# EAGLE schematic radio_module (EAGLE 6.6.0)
AUTHOR: Joshua Adkins; REV: A; TITLE: Radio Module

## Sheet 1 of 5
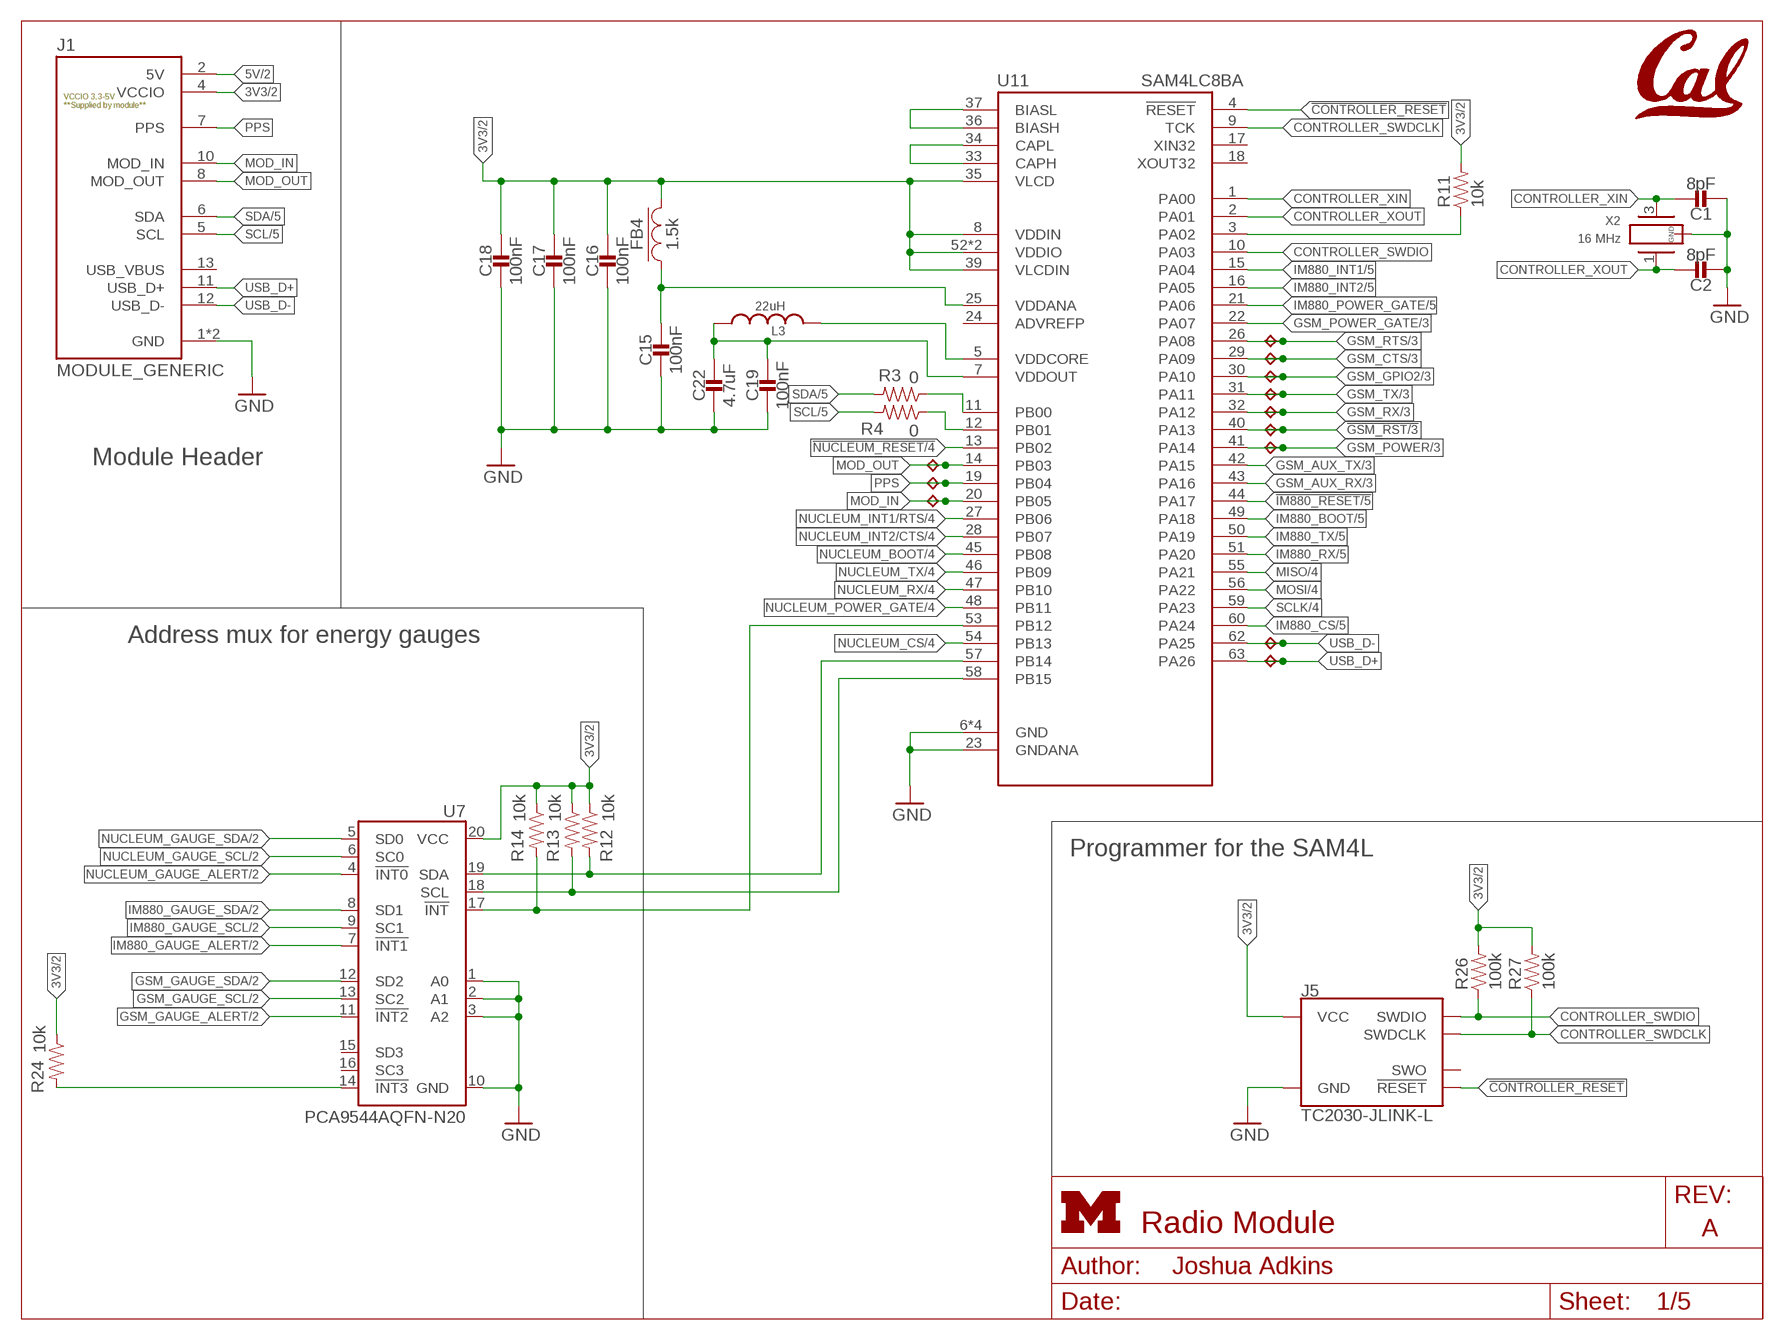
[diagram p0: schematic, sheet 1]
FRAME2 (LETTER_L_UMICH): HEIGHT: 8.5in; WIDTH: 11in

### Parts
C1  8pF  CAPACITOR0402_CAP  [0402_CAP]
C2  8pF  CAPACITOR0402_CAP  [0402_CAP]
C15  100nF  CAPACITOR0402_CAP  [0402_CAP]
C16  100nF  CAPACITOR0402_CAP  [0402_CAP]
C17  100nF  CAPACITOR0402_CAP  [0402_CAP]
C18  100nF  CAPACITOR0402_CAP  [0402_CAP]
C19  100nF  CAPACITOR0402_CAP  [0402_CAP]
C22  4.7uF  CAPACITOR0402_CAP  [0402_CAP]
FB4  1.5k  FERRITE_BEAD0402  [0402_CAP]
J1  MODULE_GENERIC  [MODULE_GENERIC]
J5  TC2030-JLINK-L  [TC2030-IDC]
L3  22uH  LHQ3NP  [1212]
R3  0  RESISTOR0402_RES  [0402_RES]
R4  0  RESISTOR0402_RES  [0402_RES]
R11  10k  RESISTOR0402_RES  [0402_RES]
R12  10k  RESISTOR0402_RES  [0402_RES]
R13  10k  RESISTOR0402_RES  [0402_RES]
R14  10k  RESISTOR0402_RES  [0402_RES]
R24  10k  RESISTOR0402_RES  [0402_RES]
R26  100k  RESISTOR0402_RES  [0402_RES]
R27  100k  RESISTOR0402_RES  [0402_RES]
TP1  TPB1,27  [B1,27]
TP2  TPB1,27  [B1,27]
TP3  TPB1,27  [B1,27]
TP4  TPB1,27  [B1,27]
TP5  TPB1,27  [B1,27]
TP6  TPB1,27  [B1,27]
TP7  TPB1,27  [B1,27]
TP8  TPB1,27  [B1,27]
TP9  TPB1,27  [B1,27]
TP10  TPB1,27  [B1,27]
TP11  TPB1,27  [B1,27]
TP12  TPB1,27  [B1,27]
U7  PCA9544AQFN-N20  [QFN-N20]
U11  SAM4LC8BA  [QFN-64-9MM]
U$1  UCB_CAL100MIL  [UCB_CAL_100MIL]
X2  16 MHz  FH1600015  [FHXXX]

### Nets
3V3: C16.1 C17.1 C18.1 FB4.2 J1.4(VCCIO) J5.1(VCC) R11.2 R12.1 R13.1 R14.1 R24.1 R26.2 R27.2 U7.20(VCC) U11.8(VDDIN) U11.35(VLCD) U11.39(VLCDIN) U11.52(VDDIO) U11.61(VDDIO) ; also sheet 2,3
5V: J1.2(5V) ; also sheet 2
!CONTROLLER_RESET: J5.3(!RESET) U11.4(!RESET)
!GSM_RST: TP7.TP U11.40(PA13) ; also sheet 3
!IM880_RESET: U11.44(PA17) ; also sheet 5
!NUCLEUM_RESET: U11.13(PB02) ; also sheet 4
CONTROLLER_BUCK/LDO_N: R11.1 U11.3(PA02)
CONTROLLER_SWDCLK: J5.4(SWDCLK) R27.1 U11.9(TCK)
CONTROLLER_SWDIO: J5.2(SWDIO) R26.1 U11.10(PA03)
CONTROLLER_XIN: C1.1 U11.1(PA00) X2.3
CONTROLLER_XOUT: C2.1 U11.2(PA01) X2.1
GND: C1.2 C2.2 C15.2 C16.2 C17.2 C18.2 C19.2 C22.2 J1.1(GND) J1.14(GND) J5.5(GND) U7.1(A0) U7.2(A1) U7.3(A2) U7.10(GND) U11.6(GND) U11.23(GNDANA) U11.38(GND) U11.64(GND) U11.GND X2.2(GND) X2.4(GND) ; also sheet 2,3,4,5
GSM_AUX_RX: U11.43(PA16) ; also sheet 3
GSM_AUX_TX: U11.42(PA15) ; also sheet 3
GSM_CTS: TP11.TP U11.29(PA09) ; also sheet 3
GSM_GAUGE_ALERT: U7.11(!INT2) ; also sheet 2
GSM_GAUGE_SCL: U7.13(SC2) ; also sheet 2
GSM_GAUGE_SDA: U7.12(SD2) ; also sheet 2
GSM_GPIO2: TP10.TP U11.30(PA10) ; also sheet 3
GSM_POWER: TP6.TP U11.41(PA14) ; also sheet 3
GSM_POWER_GATE: U11.22(PA07) ; also sheet 3
GSM_RTS: TP12.TP U11.26(PA08) ; also sheet 3
GSM_RX: TP8.TP U11.32(PA12) ; also sheet 3
GSM_TX: TP9.TP U11.31(PA11) ; also sheet 3
IM880_BOOT: U11.49(PA18) ; also sheet 5
IM880_CS: U11.60(PA24) ; also sheet 5
IM880_GAUGE_ALERT: U7.7(!INT1) ; also sheet 2
IM880_GAUGE_SCL: U7.9(SC1) ; also sheet 2
IM880_GAUGE_SDA: U7.8(SD1) ; also sheet 2
IM880_INT1: U11.15(PA04) ; also sheet 5
IM880_INT2: U11.16(PA05) ; also sheet 5
IM880_POWER_GATE: U11.21(PA06) ; also sheet 5
IM880_RX: U11.51(PA20) ; also sheet 5
IM880_TX: U11.50(PA19) ; also sheet 5
MISO: U11.55(PA21) ; also sheet 4,5
MOD_IN: J1.10(MOD_IN) TP3.TP U11.20(PB05)
MOD_OUT: J1.8(MOD_OUT) TP1.TP U11.14(PB03)
MOSI: U11.56(PA22) ; also sheet 4,5
N$9: R14.2 U7.17(!INT) U11.53(PB12)
N$12: R24.2 U7.14(!INT3)
N$17: R3.1 U11.11(PB00)
N$18: R4.1 U11.12(PB01)
N$33: C15.1 FB4.1 U11.25(VDDANA)
N$44: C19.1 C22.1 L3.P$1 U11.7(VDDOUT)
N$52: L3.P$2 U11.5(VDDCORE)
N$53: U11.36(BIASH) U11.37(BIASL)
N$54: U11.33(CAPH) U11.34(CAPL)
NUCLEUM_BOOT: U11.45(PB08) ; also sheet 4
NUCLEUM_CS: U11.54(PB13) ; also sheet 4
NUCLEUM_GAUGE_ALERT: U7.4(!INT0) ; also sheet 2
NUCLEUM_GAUGE_SCL: U7.6(SC0) ; also sheet 2
NUCLEUM_GAUGE_SDA: U7.5(SD0) ; also sheet 2
NUCLEUM_INT1/RTS: U11.27(PB06) ; also sheet 4
NUCLEUM_INT2/CTS: U11.28(PB07) ; also sheet 4
NUCLEUM_POWER_GATE: U11.48(PB11) ; also sheet 4
NUCLEUM_RX: U11.47(PB10) ; also sheet 4
NUCLEUM_TX: U11.46(PB09) ; also sheet 4
PPS: J1.7(PPS) TP2.TP U11.19(PB04)
SCL: J1.5(SCL) R4.2 ; also sheet 5
SCL_INTERNAL: R13.2 U7.18(SCL) U11.58(PB15)
SCLK: U11.59(PA23) ; also sheet 4,5
SDA: J1.6(SDA) R3.2 ; also sheet 5
SDA_INTERNAL: R12.2 U7.19(SDA) U11.57(PB14)
USB_D+: J1.11(USB_D+) TP4.TP U11.63(PA26)
USB_D-: J1.12(USB_D-) TP5.TP U11.62(PA25)
Unconnected: J1.13(USB_VBUS) J5.6(SWO) U7.15(SD3) U7.16(SC3) U11.17(XIN32) U11.18(XOUT32)

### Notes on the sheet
- Module Header
- Address mux for energy gauges
- Programmer for the SAM4L

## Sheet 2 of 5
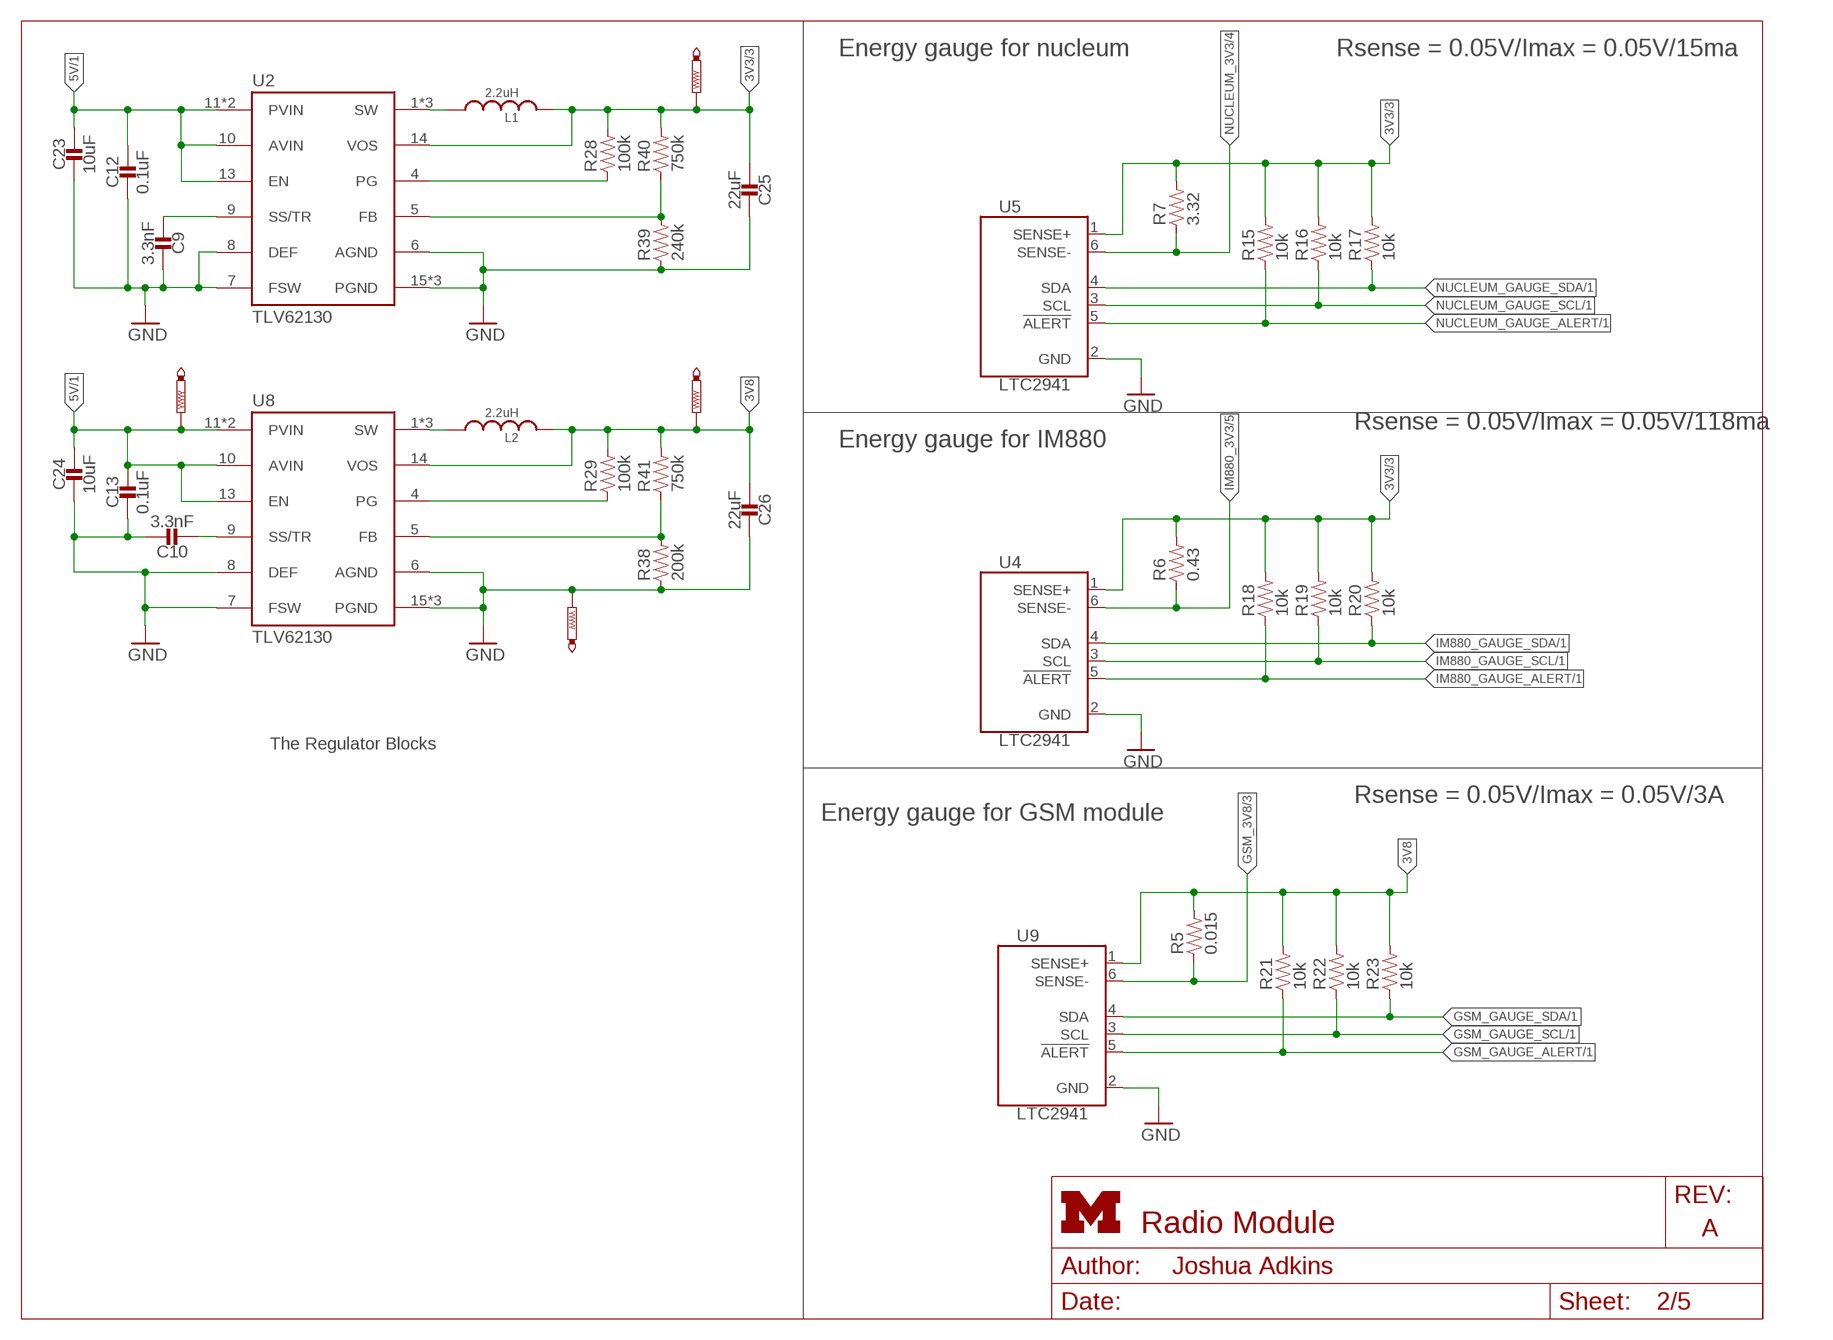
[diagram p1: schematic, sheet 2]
FRAME5 (LETTER_L_UMICH): HEIGHT: 8.5in; WIDTH: 11in

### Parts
C9  3.3nF  CAPACITOR0402_CAP  [0402_CAP]
C10  3.3nF  CAPACITOR0402_CAP  [0402_CAP]
C12  0.1uF  CAPACITOR0402_CAP  [0402_CAP]
C13  0.1uF  CAPACITOR0402_CAP  [0402_CAP]
C23  10uF  CAPACITOR0402_CAP  [0402_CAP]
C24  10uF  CAPACITOR0402_CAP  [0402_CAP]
C25  22uF  CAPACITOR0402_CAP  [0402_CAP]
C26  22uF  CAPACITOR0402_CAP  [0402_CAP]
L1  2.2uH  INDUCTORIHL  [IHL-1212BZ-11]
L2  2.2uH  INDUCTORIHL  [IHL-1212BZ-11]
R5  0.015  RESISTOR0603_RES  [0603-RES]
R6  0.43  RESISTOR0402_RES  [0402_RES]
R7  3.32  RESISTOR0402_RES  [0402_RES]
R15  10k  RESISTOR0402_RES  [0402_RES]
R16  10k  RESISTOR0402_RES  [0402_RES]
R17  10k  RESISTOR0402_RES  [0402_RES]
R18  10k  RESISTOR0402_RES  [0402_RES]
R19  10k  RESISTOR0402_RES  [0402_RES]
R20  10k  RESISTOR0402_RES  [0402_RES]
R21  10k  RESISTOR0402_RES  [0402_RES]
R22  10k  RESISTOR0402_RES  [0402_RES]
R23  10k  RESISTOR0402_RES  [0402_RES]
R28  100k  RESISTOR0402_RES  [0402_RES]
R29  100k  RESISTOR0402_RES  [0402_RES]
R38  200k  RESISTOR0402_RES  [0402_RES]
R39  240k  RESISTOR0402_RES  [0402_RES]
R40  750k  RESISTOR0402_RES  [0402_RES]
R41  750k  RESISTOR0402_RES  [0402_RES]
TP14  PTR1PAD1-13  [P1-13]
TP15  PTR1PAD1-13  [P1-13]
TP16  PTR1PAD1-13  [P1-13]
TP17  PTR1PAD1-13  [P1-13]
U2  TLV62130  [TQFN-16/3MM]
U4  LTC2941  [DFN-6-2MMX3MM]
U5  LTC2941  [DFN-6-2MMX3MM]
U8  TLV62130  [TQFN-16/3MM]
U9  LTC2941  [DFN-6-2MMX3MM]

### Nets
3V3: C25.2 L1.P$2 R6.2 R7.2 R15.2 R16.2 R17.2 R18.2 R19.2 R20.2 R28.2 R40.2 TP17.TP U2.14(VOS) U4.1(SENSE+) U5.1(SENSE+) ; also sheet 1,3
3V8: C26.2 L2.P$2 R5.2 R21.2 R22.2 R23.2 R29.2 R41.2 TP14.TP U8.14(VOS) U9.1(SENSE+)
3V8SWOUT: L2.P$1 U8.1(SW) U8.2(SW) U8.3(SW)
3VSWOUT: L1.P$1 U2.1(SW) U2.2(SW) U2.3(SW)
5V: C12.1 C13.1 C23.1 C24.1 TP16.TP U2.10(AVIN) U2.11(PVIN) U2.12(PVIN) U2.13(EN) U8.10(AVIN) U8.11(PVIN) U8.12(PVIN) U8.13(EN) ; also sheet 1
GND: C9.1 C10.1 C12.2 C13.2 C23.2 C24.2 C25.1 C26.1 R38.1 R39.1 TP15.TP U2.6(AGND) U2.7(FSW) U2.8(DEF) U2.15(PGND) U2.16(PGND) U2.GND U4.2(GND) U5.2(GND) U8.6(AGND) U8.7(FSW) U8.8(DEF) U8.15(PGND) U8.16(PGND) U8.GND U9.2(GND) ; also sheet 1,3,4,5
GSM_3V8: R5.1 U9.6(SENSE-) ; also sheet 3
GSM_GAUGE_ALERT: R21.1 U9.5(!ALERT) ; also sheet 1
GSM_GAUGE_SCL: R22.1 U9.3(SCL) ; also sheet 1
GSM_GAUGE_SDA: R23.1 U9.4(SDA) ; also sheet 1
IM880_3V3: R6.1 U4.6(SENSE-) ; also sheet 5
IM880_GAUGE_ALERT: R18.1 U4.5(!ALERT) ; also sheet 1
IM880_GAUGE_SCL: R19.1 U4.3(SCL) ; also sheet 1
IM880_GAUGE_SDA: R20.1 U4.4(SDA) ; also sheet 1
N$34: C9.2 U2.9(SS/TR)
N$36: R28.1 U2.4(PG)
N$37: R39.2 R40.1 U2.5(FB)
N$38: C10.2 U8.9(SS/TR)
N$40: R29.1 U8.4(PG)
N$41: R38.2 R41.1 U8.5(FB)
NUCLEUM_3V3: R7.1 U5.6(SENSE-) ; also sheet 4
NUCLEUM_GAUGE_ALERT: R15.1 U5.5(!ALERT) ; also sheet 1
NUCLEUM_GAUGE_SCL: R16.1 U5.3(SCL) ; also sheet 1
NUCLEUM_GAUGE_SDA: R17.1 U5.4(SDA) ; also sheet 1

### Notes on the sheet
- Energy gauge for nucleum | Rsense = 0.05V/Imax = 0.05V/15ma
- Rsense = 0.05V/Imax = 0.05V/118ma
- Energy gauge for IM880
- The Regulator Blocks
- Rsense = 0.05V/Imax = 0.05V/3A
- Energy gauge for GSM module

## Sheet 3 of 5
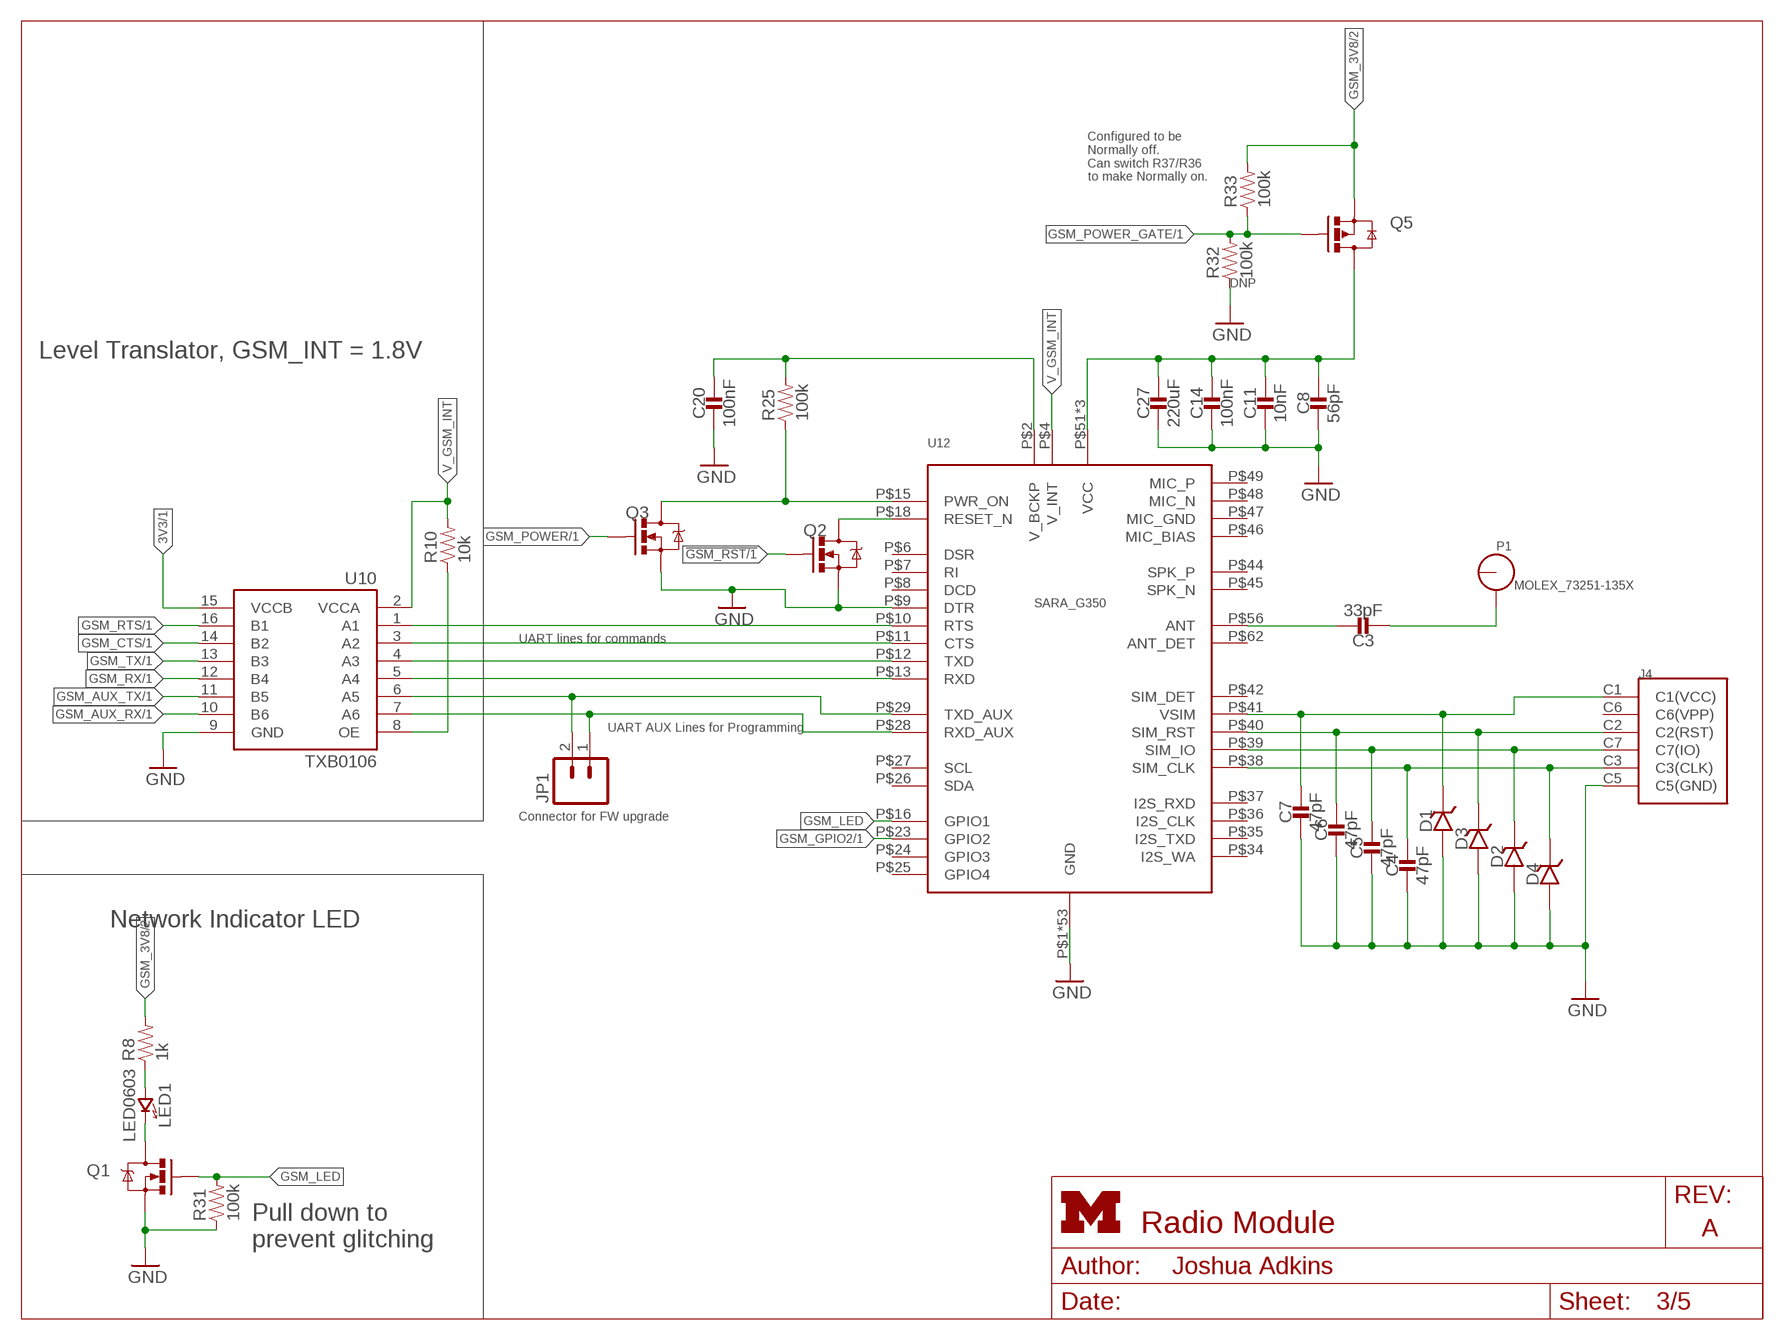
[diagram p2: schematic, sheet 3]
FRAME1 (LETTER_L_UMICH): HEIGHT: 8.5in; WIDTH: 11in

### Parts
C3  33pF  CAPACITOR0603_CAP  [0603_CAP]
C4  47pF  CAPACITOR0402_CAP  [0402_CAP]
C5  47pF  CAPACITOR0402_CAP  [0402_CAP]
C6  47pF  CAPACITOR0402_CAP  [0402_CAP]
C7  47pF  CAPACITOR0402_CAP  [0402_CAP]
C8  56pF  CAPACITOR0402_CAP  [0402_CAP]
C11  10nF  CAPACITOR0402_CAP  [0402_CAP]
C14  100nF  CAPACITOR0402_CAP  [0402_CAP]
C20  100nF  CAPACITOR0402_CAP  [0402_CAP]
C27  220uF  CAPACITOR1210_CAP  [1210_CAP]
D1  14V  DIODE_ZENER  [0402_DIODE]
D2  DIODE_ZENER  [0402_DIODE]
D3  DIODE_ZENER  [0402_DIODE]
D4  DIODE_ZENER  [0402_DIODE]
J4  NANO_SIM  [WURTH_NANO_SIM]
JP1  M02PTH  [1X02]
LED1  LED0603  [LED-0603]
P1  MOLEX_73251-135X  [SMA-J/PCB]
Q1  MOSFET-NCHANNELXFDN-3  [XFDFN-3]
Q2  MOSFET-NCHANNELXFDN-3  [XFDFN-3]
Q3  MOSFET-NCHANNELXFDN-3  [XFDFN-3]
Q5  SI223DDS  [SOT23-3]
R8  1k  RESISTOR0402_RES  [0402_RES]
R10  10k  RESISTOR0402_RES  [0402_RES]
R25  100k  RESISTOR0402_RES  [0402_RES]
R31  100k  RESISTOR0402_RES  [0402_RES]
R32  100k  RESISTOR0402_RES  [0402_RES]
R33  100k  RESISTOR0402_RES  [0402_RES]
U10  TXB0106  [R-PVQFN-N16]
U12  UBLOX_SARA_G350  [UBLOX_SARA_G3]

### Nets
3V3: U10.15(VCCB) ; also sheet 1,2
!GSM_RST: Q2.G ; also sheet 1
GND: C4.2 C5.2 C6.2 C7.2 C8.2 C11.2 C14.2 C20.2 C27.2 D1.ANODE D2.ANODE D3.ANODE D4.ANODE J4.C5(C5(GND)) Q1.S Q2.S Q3.S R31.1 R32.1 U10.9(GND) U12.P65(GND) U12.P66(GND) U12.P67(GND) U12.P68(GND) U12.P69(GND) U12.P70(GND) U12.P71(GND) U12.P72(GND) U12.P73(GND) U12.P74(GND) U12.P75(GND) U12.P76(GND) U12.P77(GND) U12.P78(GND) U12.P79(GND) U12.P80(GND) U12.P81(GND) U12.P82(GND) U12.P83(GND) U12.P84(GND) U12.P85(GND) U12.P86(GND) U12.P87(GND) U12.P88(GND) U12.P89(GND) U12.P90(GND) U12.P91(GND) U12.P92(GND) U12.P93(GND) U12.P94(GND) U12.P95(GND) U12.P96(GND) U12.P$1(GND) U12.P$3(GND) U12.P$5(GND) U12.P$9(DTR) U12.P$14(GND) U12.P$20(GND) U12.P$21(GND) U12.P$22(GND) U12.P$30(GND) U12.P$32(GND) U12.P$33(GND) U12.P$43(GND) U12.P$50(GND) U12.P$54(GND) U12.P$55(GND) U12.P$57(GND) U12.P$58(GND) U12.P$59(GND) U12.P$60(GND) U12.P$61(GND) U12.P$63(GND) U12.P$64(GND) ; also sheet 1,2,4,5
GSM_3V8: Q5.2(S) R8.2 R33.2 ; also sheet 2
GSM_AUX_RX: U10.10(B6) ; also sheet 1
GSM_AUX_TX: U10.11(B5) ; also sheet 1
GSM_CTS: U10.14(B2) ; also sheet 1
GSM_GATED: C8.1 C11.1 C14.1 C27.1 Q5.3(D) U12.P$51(VCC) U12.P$52(VCC) U12.P$53(VCC)
GSM_GPIO2: U12.P$23(GPIO2) ; also sheet 1
GSM_LED: Q1.G R31.2 U12.P$16(GPIO1)
GSM_POWER: Q3.G ; also sheet 1
GSM_POWER_GATE: Q5.1(G) R32.2 R33.1 ; also sheet 1
GSM_RTS: U10.16(B1) ; also sheet 1
GSM_RX: U10.12(B4) ; also sheet 1
GSM_TX: U10.13(B3) ; also sheet 1
N$1: C7.1 D1.CATHODE J4.C1(C1(VCC)) U12.P$41(VSIM)
N$2: C6.1 D3.CATHODE J4.C2(C2(RST)) U12.P$40(SIM_RST)
N$3: C5.1 D2.CATHODE J4.C7(C7(IO)) U12.P$39(SIM_IO)
N$4: C4.1 D4.CATHODE J4.C3(C3(CLK)) U12.P$38(SIM_CLK)
N$5: R10.1 U10.8(OE)
N$6: C3.1 U12.P$56(ANT)
N$7: C3.2 P1.2 P1.3 P1.4 P1.5
N$8: LED1.A(ANODE) R8.1
N$10: U10.4(A3) U12.P$12(TXD)
N$11: U10.5(A4) U12.P$13(RXD)
N$13: LED1.C(CATHODE) Q1.D
N$14: Q2.D U12.P$18(RESET_N)
N$15: C20.1 R25.2 U12.P$2(V_BCKP)
N$16: Q3.D R25.1 U12.P$15(PWR_ON)
N$20: JP1.2 U10.6(A5) U12.P$29(TXD_AUX)
N$21: JP1.1 U10.7(A6) U12.P$28(RXD_AUX)
N$22: U10.3(A2) U12.P$11(CTS)
N$23: U10.1(A1) U12.P$10(RTS)
V_GSM_INT: R10.2 U10.2(VCCA) U12.P$4(V_INT)
Unconnected: J4.C6(C6(VPP)) P1.1(ANT) U12.P$6(DSR) U12.P$7(RI) U12.P$8(DCD) U12.P$24(GPIO3) U12.P$25(GPIO4) U12.P$26(SDA) U12.P$27(SCL) U12.P$34(I2S_WA) U12.P$35(I2S_TXD) U12.P$36(I2S_CLK) U12.P$37(I2S_RXD) U12.P$42(SIM_DET) U12.P$44(SPK_P) U12.P$45(SPK_N) U12.P$46(MIC_BIAS) U12.P$47(MIC_GND) U12.P$48(MIC_N) U12.P$49(MIC_P) U12.P$62(ANT_DET)

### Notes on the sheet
- Configured to be
  Normally off.
  Can switch R37/R36 
  to make Normally on.
- DNP
- Level Translator, GSM_INT = 1.8V
- UART lines for commands
- UART AUX Lines for Programming
- Connector for FW upgrade
- Network Indicator LED
- Pull down to 
  prevent glitching

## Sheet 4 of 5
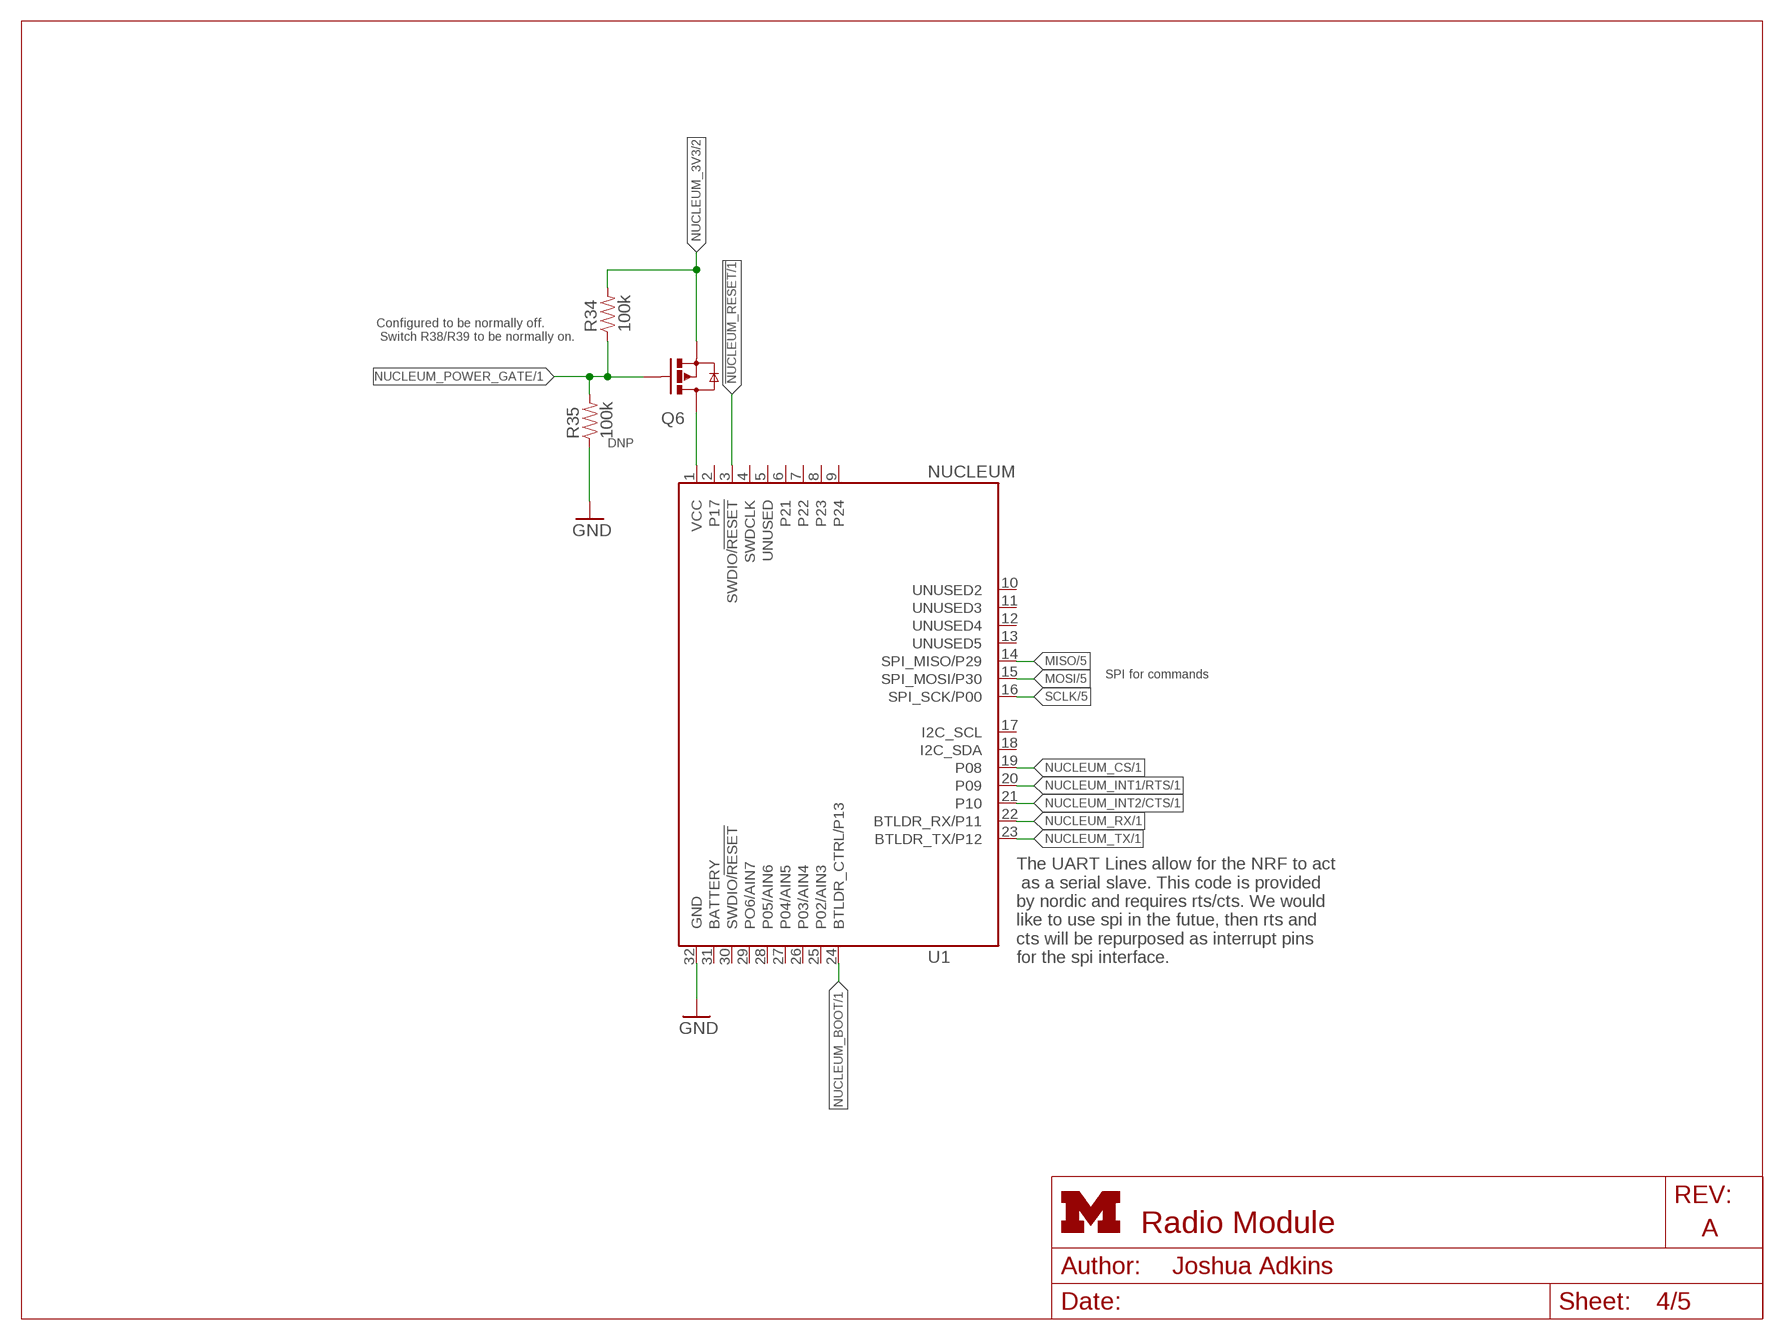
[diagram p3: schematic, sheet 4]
FRAME3 (LETTER_L_UMICH): HEIGHT: 8.5in; WIDTH: 11in

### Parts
Q6  SI223DDS  [SOT23-3]
R34  100k  RESISTOR0402_RES  [0402_RES]
R35  100k  RESISTOR0402_RES  [0402_RES]
U1  NUCLEUM  [NUCLEUM]

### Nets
!NUCLEUM_RESET: U1.3(SWDIO/!RESET) ; also sheet 1
GND: R35.1 U1.32(GND) ; also sheet 1,2,3,5
MISO: U1.14(SPI_MISO/P29) ; also sheet 1,5
MOSI: U1.15(SPI_MOSI/P30) ; also sheet 1,5
N$19: Q6.3(D) U1.1(VCC)
NUCLEUM_3V3: Q6.2(S) R34.2 ; also sheet 2
NUCLEUM_BOOT: U1.24(BTLDR_CTRL/P13) ; also sheet 1
NUCLEUM_CS: U1.19(P08) ; also sheet 1
NUCLEUM_INT1/RTS: U1.20(P09) ; also sheet 1
NUCLEUM_INT2/CTS: U1.21(P10) ; also sheet 1
NUCLEUM_POWER_GATE: Q6.1(G) R34.1 R35.2 ; also sheet 1
NUCLEUM_RX: U1.22(BTLDR_RX/P11) ; also sheet 1
NUCLEUM_TX: U1.23(BTLDR_TX/P12) ; also sheet 1
SCLK: U1.16(SPI_SCK/P00) ; also sheet 1,5
Unconnected: U1.2(P17) U1.4(SWDCLK) U1.5(UNUSED) U1.6(P21) U1.7(P22) U1.8(P23) U1.9(P24) U1.10(UNUSED2) U1.11(UNUSED3) U1.12(UNUSED4) U1.13(UNUSED5) U1.17(I2C_SCL) U1.18(I2C_SDA) U1.25(P02/AIN3) U1.26(P03/AIN4) U1.27(P04/AIN5) U1.28(P05/AIN6) U1.29(PO6/AIN7) U1.30(SWDIO/!RESET) U1.31(BATTERY)

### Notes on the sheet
- Configured to be normally off.
   Switch R38/R39 to be normally on.
- DNP
- SPI for commands
- The UART Lines allow for the NRF to act
   as a serial slave. This code is provided 
  by nordic and requires rts/cts. We would 
  like to use spi in the futue, then rts and 
  cts will be repurposed as interrupt pins 
  for the spi interface.

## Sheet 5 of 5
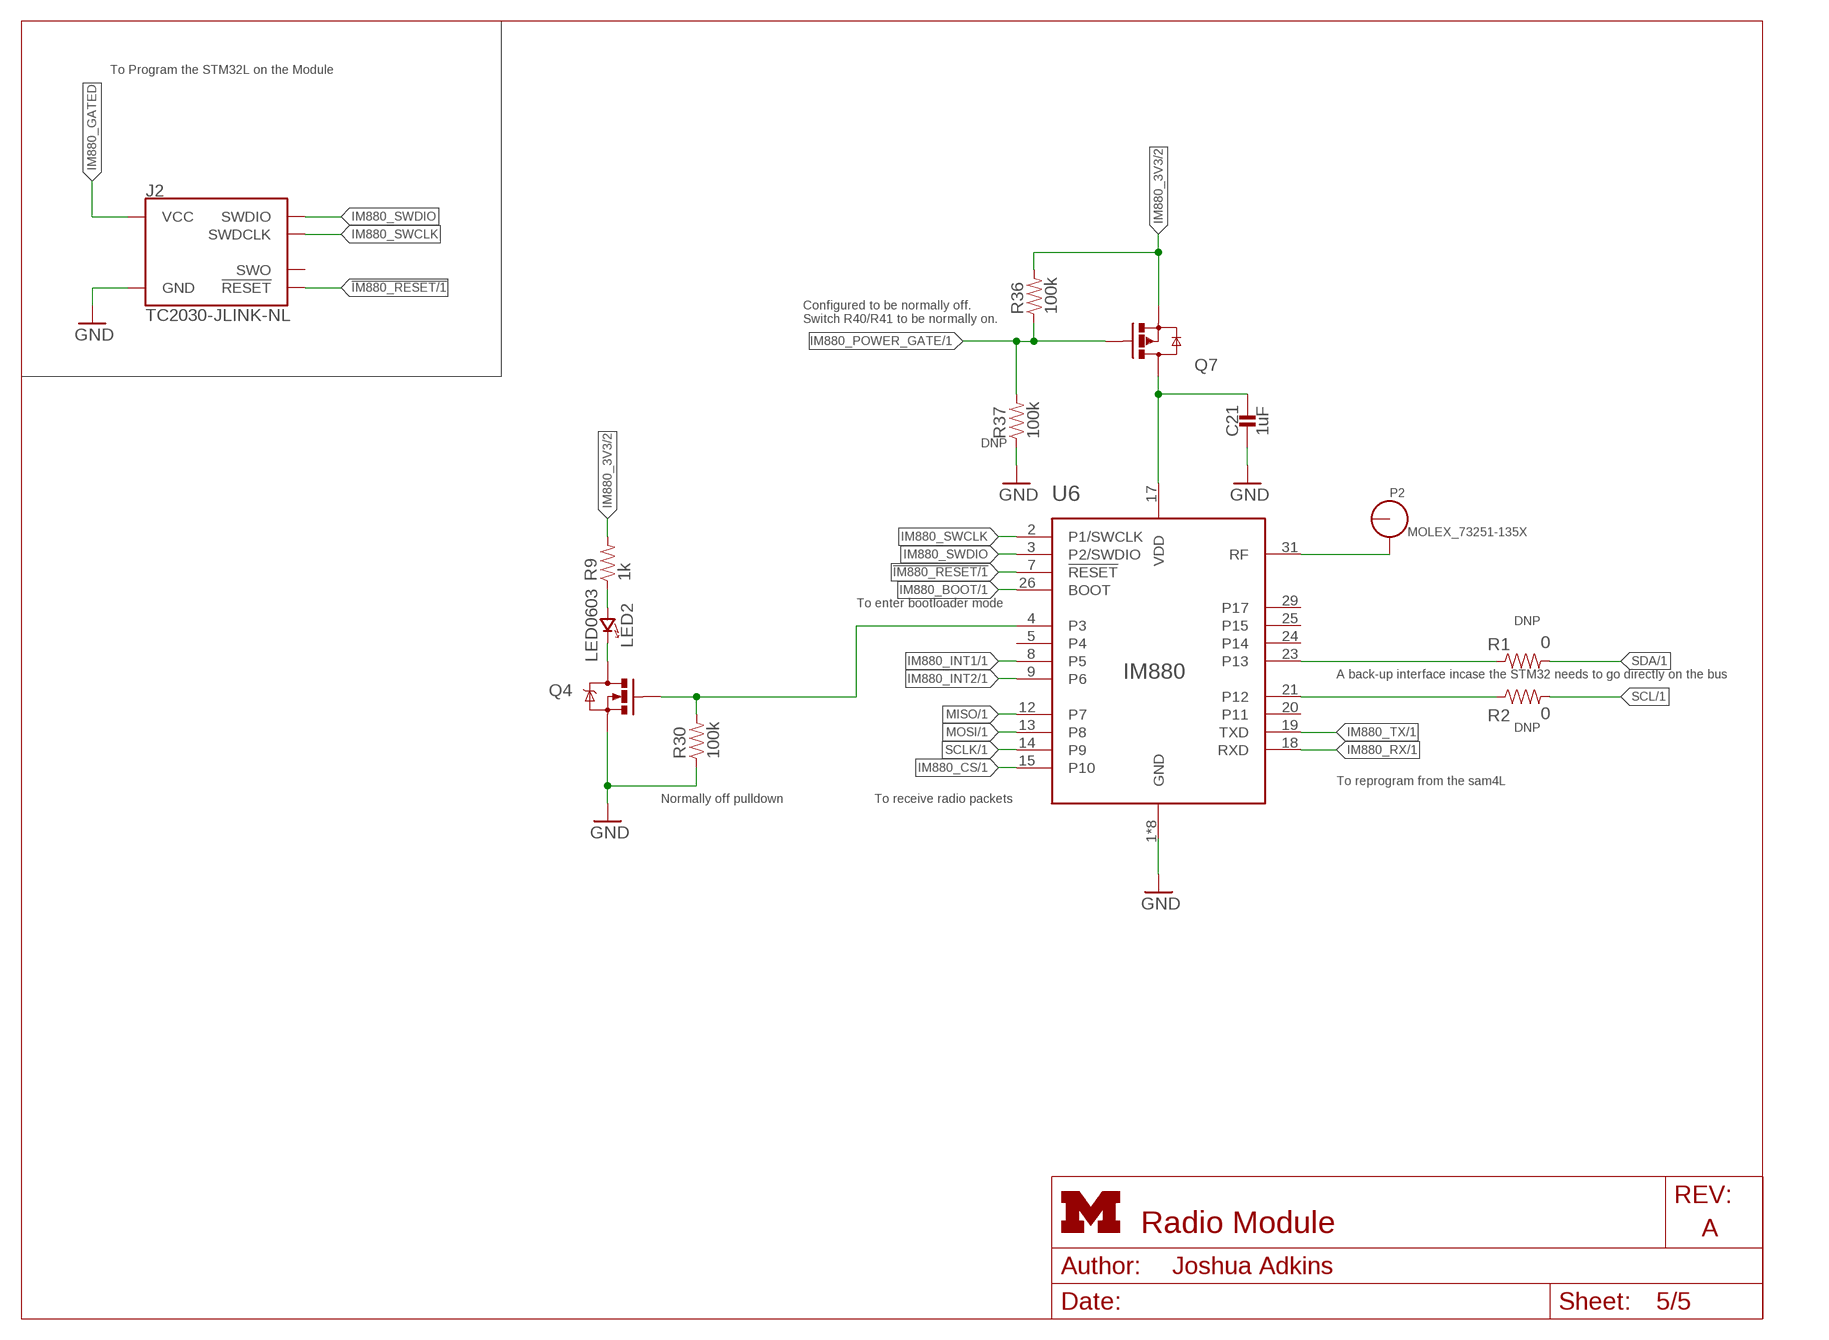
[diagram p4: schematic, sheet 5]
FRAME4 (LETTER_L_UMICH): HEIGHT: 8.5in; WIDTH: 11in

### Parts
C21  1uF  CAPACITOR0402_CAP  [0402_CAP]
J2  TC2030-JLINK-NL  [TC2030-IDC-NL]
LED2  LED0603  [LED-0603]
P2  MOLEX_73251-135X  [SMA-J/PCB]
Q4  MOSFET-NCHANNELXFDN-3  [XFDFN-3]
Q7  SI223DDS  [SOT23-3]
R1  0  RESISTOR0402_RES  [0402_RES]
R2  0  RESISTOR0402_RES  [0402_RES]
R9  1k  RESISTOR0402_RES  [0402_RES]
R30  100k  RESISTOR0402_RES  [0402_RES]
R36  100k  RESISTOR0402_RES  [0402_RES]
R37  100k  RESISTOR0402_RES  [0402_RES]
U6  IM880_MODULE  [IM880_MODULE]

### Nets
!IM880_RESET: J2.3(!RESET) U6.7(!RESET) ; also sheet 1
GND: C21.2 J2.5(GND) Q4.S R30.1 R37.1 U6.1(GND) U6.6(GND) U6.11(GND) U6.16(GND) U6.22(GND) U6.27(GND) U6.30(GND) U6.32(GND) ; also sheet 1,2,3,4
IM880_3V3: Q7.2(S) R9.2 R36.2 ; also sheet 2
IM880_BOOT: U6.26(BOOT) ; also sheet 1
IM880_CS: U6.15(P10) ; also sheet 1
IM880_GATED: C21.1 J2.1(VCC) Q7.3(D) U6.17(VDD)
IM880_INT1: U6.8(P5) ; also sheet 1
IM880_INT2: U6.9(P6) ; also sheet 1
IM880_NETWORK: Q4.G R30.2 U6.4(P3)
IM880_POWER_GATE: Q7.1(G) R36.1 R37.2 ; also sheet 1
IM880_RX: U6.18(RXD) ; also sheet 1
IM880_SWCLK: J2.4(SWDCLK) U6.2(P1/SWCLK)
IM880_SWDIO: J2.2(SWDIO) U6.3(P2/SWDIO)
IM880_TX: U6.19(TXD) ; also sheet 1
MISO: U6.12(P7) ; also sheet 1,4
MOSI: U6.13(P8) ; also sheet 1,4
N$25: R1.1 U6.23(P13)
N$26: R2.1 U6.21(P12)
N$27: LED2.A(ANODE) R9.1
N$28: LED2.C(CATHODE) Q4.D
N$29: P2.2 P2.3 P2.4 P2.5 U6.31(RF)
SCL: R2.2 ; also sheet 1
SCLK: U6.14(P9) ; also sheet 1,4
SDA: R1.2 ; also sheet 1
Unconnected: J2.6(SWO) P2.1(ANT) U6.5(P4) U6.20(P11) U6.24(P14) U6.25(P15) U6.29(P17)

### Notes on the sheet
- To Program the STM32L on the Module
- Configured to be normally off.
  Switch R40/R41 to be normally on.
- DNP
- To enter bootloader mode
- DNP
- A back-up interface incase the STM32 needs to go directly on the bus
- DNP
- To reprogram from the sam4L
- Normally off pulldown | To receive radio packets

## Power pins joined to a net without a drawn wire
ADVREFP: U11.24(ADVREFP)

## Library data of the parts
C1 C2 = passives:CAPACITOR: 0402 Capacitor; DIGIKEY: 490-8230-1-ND
C3-C14 C20 C21 C23-C27 = passives:CAPACITOR: 0402 Capacitor
C15-C19 = passives:CAPACITOR: 0402 Capacitor; DIGIKEY: 490-10777-1-ND
C22 = passives:CAPACITOR: 0402 Capacitor; DIGIKEY: 490-13252-1-ND
D1-D4 = passives:DIODE_ZENER
FB4 = passives:FERRITE_BEAD; DIGIKEY: 490-5216-1-ND
J1 = signpost:MODULE_GENERIC: Module header and PCB guildes for signposts; DIGIKEY: S9170-ND
J2 J5 = connector:TC2030-JLINK
J4 = signpost:NANO_SIM: WURTH Nano SIM Connector; DIGIKEY: 732-5954-1-ND
JP1 = SparkFun-Connectors:M02: Header 2
L1 L2 = passives:INDUCTOR: A very specific inductor; DIGIKEY: 541-1322-1-ND
L3 = signpost:LHQ3NP: LHQ3NP Inductor; DIGIKEY: 490-5350-1-ND
LED1 LED2 = leds:LED: LED
P1 P2 = connector:MOLEX_73251-135X: SMA JACK SMT 50 OHM; DIGIKEY: WM9357-ND
Q1-Q4 = fets:MOSFET-NCHANNEL: Generic NMOS footprint; DIGIKEY: DMN2400UFB4-7DICT-ND
Q5-Q7 = fets:SI223DDS: 6A SOT-23 P Fet; DIGIKEY: SI2333DDS-T1-GE3CT-ND
R1 R2 R5-R10 R15-R23 R25 R28-R41 = passives:RESISTOR: Resistor
R3 R4 R11-R14 R24 = passives:RESISTOR: Resistor; DIGIKEY: 1276-3431-1-ND
R26 R27 = passives:RESISTOR: Resistor; DIGIKEY: 1276-3432-1-ND
TP1-TP12 = testpad:TP: Test pad
TP14-TP17 = testpad:PTR1: TEST PIN
U1 = nucleum:NUCLEUM: Nucleum sensorboard prototyping module.
U2 U8 = chips:TLV62130: High Efficient 3A switching step-down regulator. 1V-5V out, 4V-17V in.; DIGIKEY: 296-35978-1-ND
U4 U5 U9 = signpost:LTC2941: I2C Battery Gas Gauge with External Sense Resistor; DIGIKEY: LTC2941IDCB#TRMPBFCT-ND
U6 = chips:IM880_MODULE: Lora Radio module by IMST
U7 = signpost:PCA9544A: 1-4 I2C/SMBUS Multiplexer with interrupt for power supply coulomb counters; DIGIKEY: 296-20960-1-ND
U10 = chips:TXB0106: 6 channel level translator; DIGIKEY: 296-23868-2-ND
U11 = chips:SAM4LC8BA: SAM4L Microcontroller. 64QFN Package. 512 Flash.; DIGIKEY: ATSAM4LC8BA-MURDKR-ND
U12 = signpost:UBLOX_SARA_G350: Sara G350 2.5G Radio Module
U$1 = logos:UCB_CAL
X2 = crystals:FH1600015: Pericom Type FH 16 MHz 2.5 x 2.0 mm; DIGIKEY: FH1600015CT-ND

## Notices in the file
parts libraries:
SparkFun-Connectors: Licensing: CC v3.0 Share-Alike You are welcome to use this library for commercial purposes.
